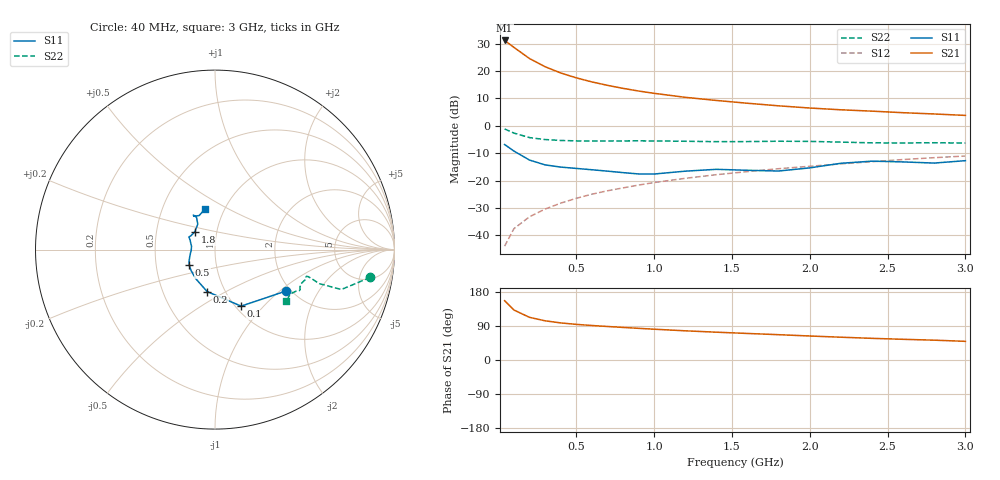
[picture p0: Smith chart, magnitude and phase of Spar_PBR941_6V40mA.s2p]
! Filename:  PBR941R.S2P  Version:  3.0
! NXP part #:  PBR941  Date: July 1998
! Bias condition:  Vce=6V, Ic=40mA
#  MHz  S  MA  R 50
! Freq  S11  S21  S12  S22
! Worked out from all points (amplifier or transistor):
!   21 points, 40 MHz to 3 GHz, reference 50 ohm
!   highest |S21| = 31.2 dB at 40 MHz (marker M1)
!   |S21| within 3 dB of that: start of sweep to 111.4 MHz
!   unconditionally stable (mu >= 1): 300.7 MHz to 2.386 GHz
!   at 300 MHz: K = 1.00, MSG = 26.0 dB, |S12| = -30.4 dB
!   at 1 GHz: K = 1.08, MAG = 14.5 dB, |S12| = -20.7 dB
!   at 3 GHz: K = 0.98, MSG = 7.4 dB, |S12| = -11.0 dB
!   lowest NFmin = 3.26 dB at 900 MHz
!   S11 on the Smith chart (normalised r, x): 40 MHz: 1.88, -1.10; 100 MHz: 1.06, -0.76; 200 MHz: 0.82, -0.41; 500 MHz: 0.74, -0.13; 1.8 GHz: 0.78, +0.16; 3 GHz: 0.81, +0.39
40  0.4568 -30.4  36.27 156.4  0.00637 75.9  0.8786 -10.1
100  0.347 -65.2  27.08 131.9  0.01331 72.9  0.7385 -17.5
200  0.2376 -100.7  16.95 112.5  0.02192 72.2  0.6113 -18.1
300  0.1941 -123.8  12.03 103.4  0.03029 76.5  0.5632 -16.8
400  0.177 -139.0  9.254 97.9  0.03884 78.0  0.5419 -16.2
500  0.1673 -149.1  7.537 94.0  0.04759 79.6  0.5323 -16.2
600  0.1583 -156.0  6.358 91.1  0.05656 80.4  0.5294 -16.5
700  0.1492 -161.8  5.501 88.5  0.06529 81.1  0.5295 -16.9
800  0.1402 -169.6  4.846 86.0  0.07373 81.6  0.5321 -17.3
900  0.1326 -178.5  4.332 83.6  0.08304 81.7  0.5329 -17.8
1000  0.1322 171.9  3.93 81.3  0.09237 81.7  0.5315 -18.3
1200  0.149 159.0  3.324 77.0  0.1103 81.4  0.5239 -19.6
1400  0.1611 154.3  2.913 73.4  0.1285 81.0  0.5153 -21.7
1600  0.1546 150.0  2.59 70.1  0.1463 80.8  0.5172 -23.7
1800  0.1499 138.5  2.324 66.8  0.1653 80.4  0.5242 -25.2
2000  0.1712 124.0  2.119 63.3  0.1831 79.6  0.5212 -26.1
2200  0.2075 119.8  1.967 60.2  0.2025 78.7  0.5051 -27.4
2400  0.2272 122.1  1.858 57.1  0.2219 77.9  0.4903 -30.0
2600  0.2199 122.5  1.741 54.6  0.2431 77.3  0.4874 -33.0
2800  0.2095 115.0  1.649 52.3  0.2628 76.3  0.4924 -35.1
3000  0.2317 103.8  1.553 49.2  0.2818 75.1  0.4863 -35.9
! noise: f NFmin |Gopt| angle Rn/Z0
500  3.305  0.152  -161.6  0.252
900  3.262  0.594  -149.7  0.074
1000  3.717  0.265  -142.7  0.298
2000  4.767  0.387  -108.2  0.774
